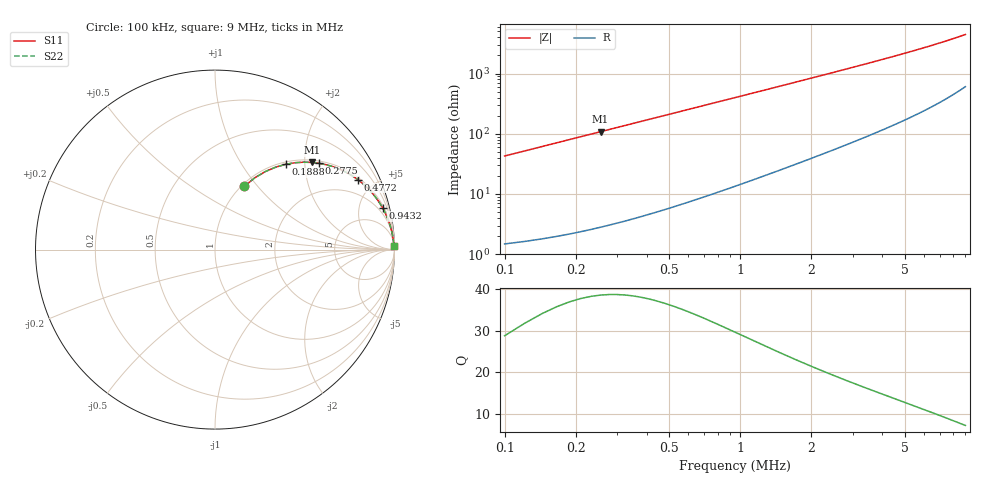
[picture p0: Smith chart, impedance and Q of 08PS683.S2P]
! Coilcraft 0805PS-683 Power Chip Inductor
! 5 February 2003
# MHZ S MA R 50
!Freq  MagS11  AngS11  MagS21  AngS21  MagS12  AngS12  MagS22  AngS22
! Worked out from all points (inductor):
!   403 points, 100 kHz to 9 MHz, reference 50 ohm
!   read as one part in series: L = 67.6 uH near 144.4 kHz
!   highest Q = 38.4 at 255.3 kHz (marker M1), where L = 67.5 uH
!   S11 on the Smith chart (normalised r, x): 100 kHz: 1.03, +0.85; 188.8 kHz: 1.04, +1.60; 277.5 kHz: 1.06, +2.35; 477.2 kHz: 1.11, +4.03; 943.2 kHz: 1.27, +7.92; 9 MHz: 13, +88
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0.1  0.3883 65.2  0.9082 -22.8  0.9082 -22.8  0.3883 65.2
0.14438  0.5173 57.2  0.8408 -31.1  0.8408 -31.1  0.5173 57.2
0.18876  0.6178 50.3  0.7698 -38.1  0.7698 -38.1  0.6178 50.3
0.25533  0.7254 42.0  0.6698 -46.5  0.6698 -46.5  0.7254 42.0
0.27752  0.7524 39.7  0.6396 -48.8  0.6396 -48.8  0.7524 39.7
0.3219  0.7965 35.7  0.5844 -52.8  0.5844 -52.8  0.7965 35.7
0.36628  0.8303 32.4  0.536 -56.1  0.536 -56.1  0.8303 32.4
0.41066  0.8566 29.6  0.4936 -58.9  0.4936 -58.9  0.8566 29.6
0.47723  0.8861 26.1  0.4399 -62.3  0.4399 -62.3  0.8861 26.1
0.56599  0.9131 22.5  0.3827 -65.9  0.3827 -65.9  0.9131 22.5
0.67694  0.9349 19.1  0.328 -69.1  0.328 -69.1  0.9349 19.1
0.94322  0.962 14.0  0.2427 -74.0  0.2427 -74.0  0.962 14.0
1.23169  0.975 10.9  0.1885 -77.0  0.1885 -77.0  0.975 10.9
1.58673  0.9829 8.5  0.1475 -79.1  0.1475 -79.1  0.9829 8.5
1.89739  0.9867 7.1  0.1238 -80.3  0.1238 -80.3  0.9867 7.1
2.25243  0.9894 6.0  0.1044 -81.2  0.1044 -81.2  0.9894 6.0
3.07346  0.9927 4.4  0.07622 -82.3  0.07622 -82.3  0.9927 4.4
3.76135  0.9941 3.5  0.06183 -82.7  0.06183 -82.7  0.9941 3.5
4.56019  0.995 2.9  0.05039 -82.9  0.05039 -82.9  0.995 2.9
6.04692  0.996 2.1  0.0368 -82.7  0.0368 -82.7  0.996 2.1
7.53365  0.9965 1.6  0.02825 -82.1  0.02825 -82.1  0.9965 1.6
9  0.9967 1.3  0.02234 -80.9  0.02234 -80.9  0.9967 1.3
